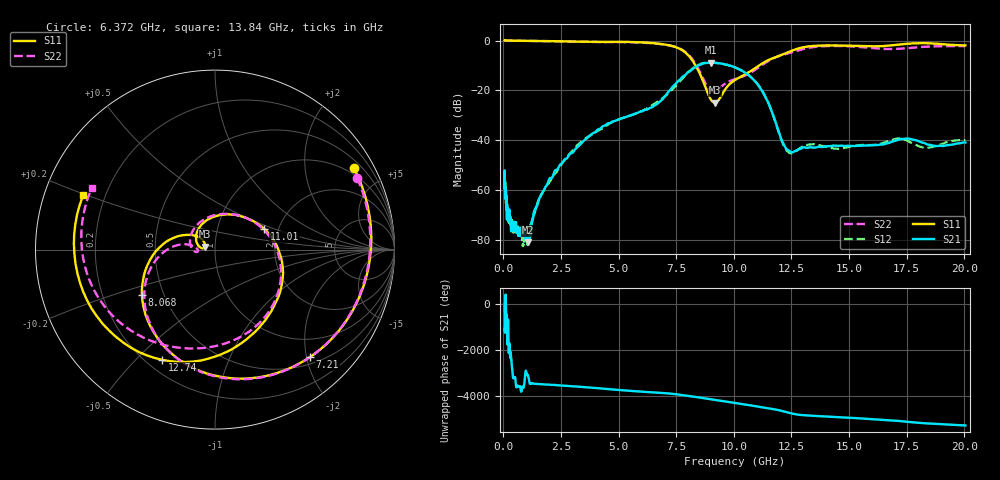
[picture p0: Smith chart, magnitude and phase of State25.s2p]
# Hz S DB R 50
!freq MagS11 AngS11 MagS21 AngS21 MagS12 AngS12 MagS22 AngS22
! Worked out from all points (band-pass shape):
!   1601 points, 50 MHz to 20.05 GHz, reference 50 ohm
!   highest |S21| = -8.88 dB at 8.994 GHz (marker M1); lowest = -81.1 dB at 1.079 GHz (marker M2)
!   |S21| within 3 dB of the highest: 8.156 GHz to 10.3 GHz (2.147 GHz wide, 23.3 % of centre)
!   lowest |S11| = -24.9 dB at 9.164 GHz (marker M3), VSWR 1.12, Z = 44.9 + j1.53 ohm
!   |S11| at or under -10 dB: 8.336 GHz to 11.09 GHz (2.756 GHz wide, 28.4 % of centre)
!   |S22| runs from -20.4 to 0.0 dB; largest |S21 - S12| = 0.022
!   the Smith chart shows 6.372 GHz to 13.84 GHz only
!   S11 on the Smith chart (normalised r, x): 6.372 GHz: 0.75, +3.51; 7.21 GHz: 0.62, -2.06; 8.068 GHz: 0.38, -0.25; 11.01 GHz: 1.69, +0.43; 12.74 GHz: 0.26, -0.60; 13.84 GHz: 0.12, +0.20
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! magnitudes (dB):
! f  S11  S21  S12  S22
! 50 MHz  0.0  -54.2  -53.7  0.0
! 135.9 MHz  0.0  -66.4  -66.2  0.0
! 149.9 MHz  0.0  -70.8  -67.6  0.0
! 163.3 MHz  0.0  -66.7  -67.9  0.0
! 220.4 MHz  0.0  -72.5  -72.5  0.0
! 251.3 MHz  0.0  -68.7  -70.7  0.0
! 369.6 MHz  0.0  -74.1  -74.1  0.0
! 1.005 GHz  -0.1  -80.3  -79.6  -0.1
! 1.079 GHz  -0.1  -81.1  -81.5  -0.1
! 1.529 GHz  -0.2  -64.0  -64.1  -0.2
! 2.722 GHz  -0.3  -47.5  -47.3  -0.4
! 6.372 GHz  -0.9  -27.0  -26.4  -1.0
! 7.21 GHz  -1.9  -20.1  -20.7  -2.0
! 7.402 GHz  -2.4  -18.0  -18.9  -2.4
! 8.068 GHz  -6.4  -12.4  -12.4  -6.0
! 8.994 GHz  -23.6  -8.9  -8.8  -20.1
! 9.164 GHz  -24.9  -8.9  -8.9  -20.4
! 11.01 GHz  -10.5  -17.4  -17.3  -11.2
! 12.23 GHz  -5.2  -42.8  -43.3  -5.5
! 12.74 GHz  -3.3  -44.0  -44.2  -4.1
! 13.84 GHz  -2.0  -42.8  -42.3  -2.3
! 20.05 GHz  -2.0  -41.0  -40.0  -2.2
